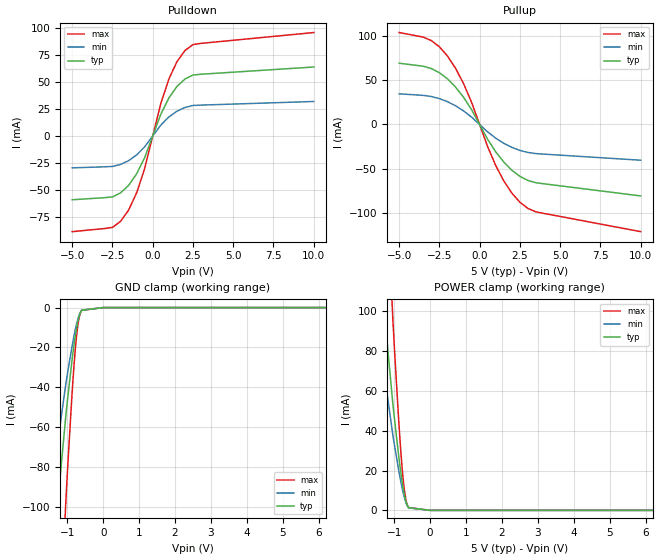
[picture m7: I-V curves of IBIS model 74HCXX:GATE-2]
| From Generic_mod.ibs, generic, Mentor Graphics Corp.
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[Model]   74HCXX:GATE-2
Model_type   I/O
Polarity   Non-Inverting
Vinl  =   0.800V
Vinh  =   2.000V
Vmeas =   1.500V
Cref  =  50.000pF
Rref  =   1.000kOhm
Vref  =   0.000V
|   typ   min   max
C_comp   5.000pF   2.500pF   7.500pF
[Voltage Range]   5.000V   4.500V   5.500V
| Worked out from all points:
|   slope of the pulldown table from 0 to 0.75 V, typ, clamps not added: 27.3 ohm
|   slope of the pullup table from 0 to 0.75 V, typ, clamps not added: 31.7 ohm
[Pulldown]
| Voltage   I(typ)   I(min)   I(max)
-5V       -58.87mA   -29.43mA   -88.3mA
-2.5V     -56.24mA   -28.12mA   -84.36mA
-2V       -52.53mA   -26.27mA   -78.8mA
-1.5V     -45.63mA   -22.82mA   -68.45mA
-1V       -34.98mA   -17.49mA   -52.47mA
-500mV    -20mA      -10mA      -30mA
500mV     20mA       10mA       30mA
1V        34.98mA    17.49mA    52.47mA
1.5V      45.63mA    22.82mA    68.45mA
2V        52.53mA    26.27mA    78.8mA
3V        56.97mA    28.48mA    85.45mA
10V       63.63mA    31.82mA    95.45mA
[Pullup]
| Voltage   I(typ)   I(min)   I(max)
-5V       68.9mA     34.45mA    103.3mA
-3V       62.89mA    31.45mA    94.33mA
-2V       51.38mA    25.69mA    77.06mA
-1.5V     42.23mA    21.12mA    63.35mA
-1V       30.7mA     15.35mA    46.05mA
-500mV    16.67mA    8.333mA    25mA
500mV     -16.67mA   -8.333mA   -25mA
1V        -30.7mA    -15.35mA   -46.05mA
1.5V      -42.23mA   -21.12mA   -63.35mA
2.5V      -58.23mA   -29.11mA   -87.34mA
3.5V      -65.46mA   -32.73mA   -98.19mA
10V       -80.28mA   -40.14mA   -120.4mA
[GND Clamp]
| Voltage   I(typ)   I(min)   I(max)
-5V       -820mA     -549.2mA   -1.627A
-1.036V   -53.26mA   -37.7mA    -95.41mA
-984.1mV  -44.54mA   -31.82mA   -78.32mA
-874.8mV  -27.32mA   -20.14mA   -45.09mA
-822.5mV  -19.88mA   -15.03mA   -31.19mA
-775.2mV  -13.87mA   -10.82mA   -20.4mA
-735.6mV  -9.524mA   -7.699mA   -13.05mA
-678.8mV  -4.762mA   -4.11mA    -5.792mA
-653.9mV  -3.293mA   -2.932mA   -3.809mA
-601.6mV  -1.347mA   -1.27mA    -1.438mA
0V        0A         0A         0A
10V       0A         0A         0A
[POWER Clamp]
| Voltage   I(typ)   I(min)   I(max)
-5V       820mA      549.2mA    1.627A
-1.036V   53.26mA    37.7mA     95.41mA
-984.1mV  44.54mA    31.82mA    78.32mA
-874.8mV  27.32mA    20.14mA    45.09mA
-822.5mV  19.88mA    15.03mA    31.19mA
-775.2mV  13.87mA    10.82mA    20.4mA
-735.6mV  9.524mA    7.699mA    13.05mA
-678.8mV  4.762mA    4.11mA     5.792mA
-653.9mV  3.293mA    2.932mA    3.809mA
-601.6mV  1.347mA    1.27mA     1.438mA
0V        0A         0A         0A
10V       0A         0A         0A
[Ramp]
|   typ   min   max
dV/dt_r   1.646V/3.600ns   0.935V/6.480ns   2.189V/2.640ns
dV/dt_f   1.637V/3.600ns   0.856V/6.480ns   2.230V/2.640ns
R_load =  50.000Ohm
|------------------- End of 74HCXX:GATE-2 -------------------------------------
